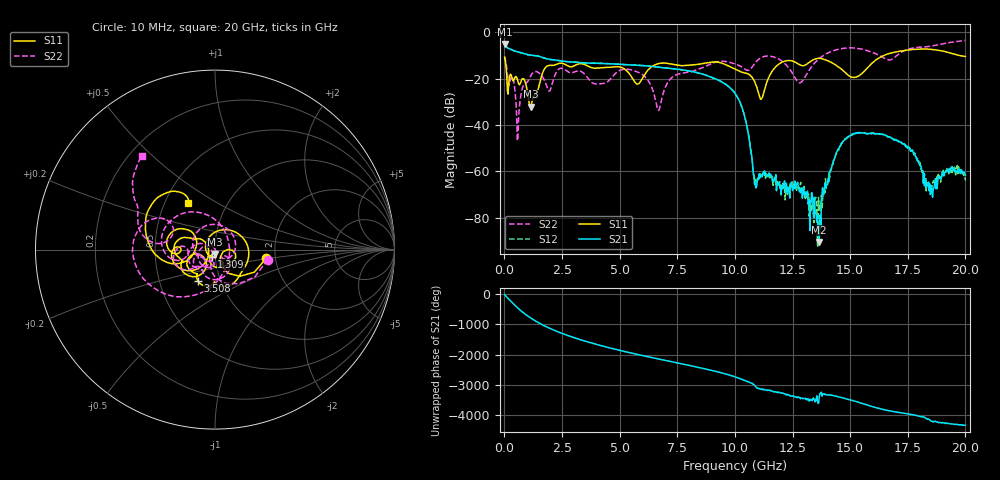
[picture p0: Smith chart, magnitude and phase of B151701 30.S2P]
!  2-Port S-parameters saved by WinCal
! VAR MeasName=S-Parameters (CALIBRATED_DATA) read from VNA (N5244A)
! VAR MeasDate=2015-12-24 19:12:45
! VAR NAME=B151701 30
! VAR FILENAME=B151701 30.S2P
! VAR DATE=2015-12-24 19:12:45
! VAR PHYS_PORTS=1,3
# Hz S DB R 50
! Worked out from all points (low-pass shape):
!   801 points, 10 MHz to 20 GHz, reference 50 ohm
!   highest |S21| = -5.14 dB at 10 MHz (marker M1); lowest = -90.3 dB at 13.65 GHz (marker M2)
!   |S21| within 3 dB of the highest: start of sweep to 453.4 MHz
!   lowest |S11| = -32.1 dB at 1.134 GHz (marker M3), VSWR 1.05, Z = 49.7 - j2.45 ohm
!   |S11| at or under -10 dB: start of sweep to 16.47 GHz; 19.71 GHz to end of sweep
!   |S22| runs from -46.7 to -3.6 dB; largest |S21 - S12| = 0.0026
!   S11 on the Smith chart (normalised r, x): 10 MHz: 1.78, -0.19; 1.309 GHz: 0.96, -0.08; 3.508 GHz: 0.78, -0.28; 20 GHz: 0.66, +0.37
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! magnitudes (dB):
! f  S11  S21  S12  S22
! 10 MHz  -10.8  -5.1  -5.1  -10.5
! 584.7 MHz  -21.0  -8.5  -8.5  -46.7
! 1.134 GHz  -32.1  -9.9  -9.9  -19.0
! 1.309 GHz  -27.1  -10.1  -10.1  -17.0
! 1.859 GHz  -14.6  -11.5  -11.5  -23.8
! 3.358 GHz  -13.6  -13.2  -13.2  -17.1
! 3.508 GHz  -14.0  -13.3  -13.3  -18.4
! 5.807 GHz  -22.3  -14.3  -14.3  -17.3
! 6.682 GHz  -13.6  -15.1  -15.1  -33.7
! 7.381 GHz  -14.0  -15.8  -15.8  -18.7
! 10.01 GHz  -15.9  -26.3  -26.3  -13.7
! 10.45 GHz  -17.6  -37.5  -37.5  -16.0
! 10.9 GHz  -22.5  -67.0  -66.0  -12.9
! 11.15 GHz  -28.7  -61.6  -61.4  -10.9
! 12.8 GHz  -14.0  -68.7  -67.6  -21.8
! 13.35 GHz  -12.1  -69.7  -75.5  -14.5
! 13.65 GHz  -11.3  -90.3  -76.6  -11.5
! 14.7 GHz  -16.6  -46.9  -46.9  -7.0
! 16.68 GHz  -9.2  -45.1  -45.0  -12.0
! 17.75 GHz  -7.4  -52.3  -51.7  -6.8
! 18.53 GHz  -7.4  -66.1  -69.1  -6.0
! 20 GHz  -10.5  -61.6  -63.9  -3.6
